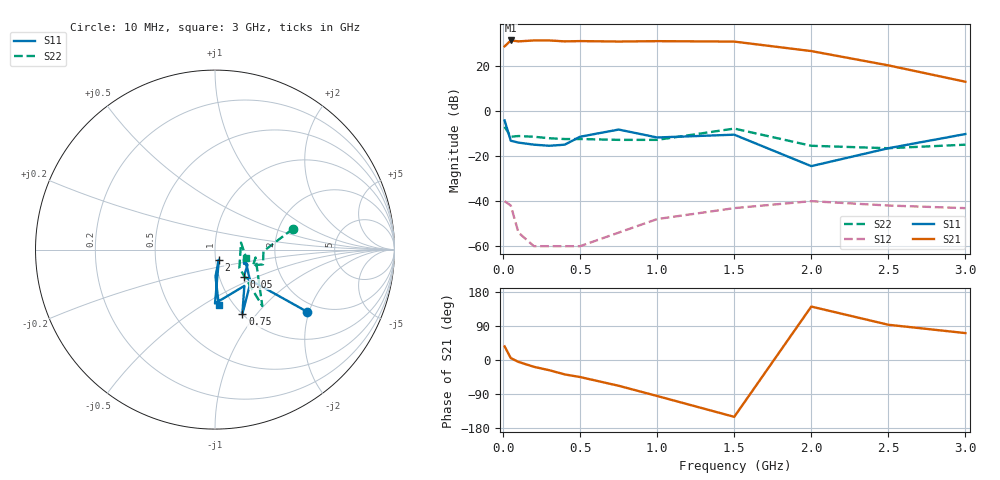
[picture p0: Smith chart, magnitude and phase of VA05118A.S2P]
!  IVA-05118  S PARAMETERS
!  Full Gain S PARAMETERS (VGC=0)!  LAST UPDATED 07-22-92
# ghz s ma r 50
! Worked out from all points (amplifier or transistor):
!   13 points, 10 MHz to 3 GHz, reference 50 ohm
!   highest |S21| = 31.4 dB at 50 MHz (marker M1)
!   |S21| within 3 dB of that: start of sweep to 1.796 GHz
!   unconditionally stable (mu >= 1): 17.87 MHz to end of sweep
!   at 100 MHz: K = 6.23, MAG = 31.6 dB, |S12| = -54.0 dB
!   at 500 MHz: K = 12.19, MAG = 31.7 dB, |S12| = -60.0 dB
!   at 3 GHz: K = 13.86, MAG = 13.7 dB, |S12| = -43.1 dB
!   S11 on the Smith chart (normalised r, x): 10 MHz: 1.73, -1.95; 50 MHz: 1.31, -0.41; 750 MHz: 1.00, -0.85; 2 GHz: 1.04, -0.12; 3 GHz: 0.86, -0.59
0.01  0.62 -34.0  27.5 36.0  0.01 -52.0  0.45 15.0
0.05  0.22 -43.0  37.2 5.0  0.008 9.0  0.27 -2.0
0.1  0.2 -25.0  35.5 -5.0  0.002 -91.0  0.28 -17.0
0.2  0.18 -26.0  37.2 -18.0  0.001 18.0  0.27 -18.0
0.3  0.17 -19.0  37.2 -27.0  0.001 91.0  0.25 -20.0
0.4  0.18 -19.0  35.5 -38.0  0.001 88.0  0.24 -22.0
0.5  0.27 -43.0  36 -45.0  0.001 101.0  0.24 -23.0
0.75  0.39 -67.0  35.2 -68.0  0.002 151.0  0.23 -23.0
1  0.26 -51.0  35.9 -95.0  0.004 116.0  0.23 -11.0
1.5  0.3 -90.0  35.1 -150.0  0.007 84.0  0.41 -50.0
2  0.06 -69.0  21.6 141.0  0.01 113.0  0.17 -37.0
2.5  0.15 -89.0  10.4 93.0  0.008 117.0  0.15 15.0
3  0.31 -86.0  4.5 71.0  0.007 136.0  0.18 -15.0
